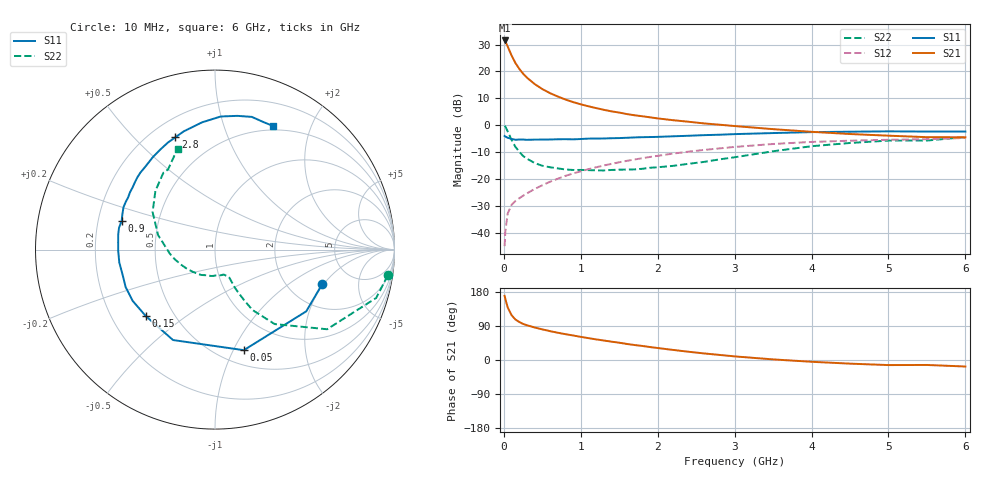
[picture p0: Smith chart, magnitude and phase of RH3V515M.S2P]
! SIEMENS Small Signal Semiconductors
! BFR106
! Si NPN RF Bipolar Junction Transistor in SOT23
! VCE = 3.5 V  IC = 15 mA
! Common Emitter S-Parameters:  August  1996
# GHz  S  MA  R  50
!  f  S11  S21  S12  S22
! GHz  MAG  ANG  MAG  ANG  MAG  ANG  MAG  ANG
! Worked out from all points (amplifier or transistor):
!   36 points, 10 MHz to 6 GHz, reference 50 ohm
!   highest |S21| = 31.5 dB at 10 MHz (marker M1)
!   |S21| within 3 dB of that: start of sweep to 61.44 MHz
!   unconditionally stable (mu >= 1): 413.1 MHz to 2.169 GHz; 5.31 GHz to end of sweep
!   at 250 MHz: K = 0.82, MSG = 22.7 dB, |S12| = -26.3 dB
!   at 1.4 GHz: K = 1.08, MAG = 8.0 dB, |S12| = -14.4 dB
!   at 6 GHz: K = 1.01, MAG = -0.3 dB, |S12| = -4.8 dB
!   S11 on the Smith chart (normalised r, x): 10 MHz: 3.07, -1.93; 50 MHz: 0.65, -1.10; 150 MHz: 0.35, -0.36; 900 MHz: 0.30, +0.14; 2.8 GHz: 0.30, +0.67; 6 GHz: 0.45, +1.47
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0.01  0.6281 -17.6  37.68 169.4  0.0056 84.1  0.9732 -8.5
0.02  0.6138 -34.1  36.13 160.9  0.0107 78.1  0.9376 -16.7
0.05  0.5829 -74.0  29.11 138.8  0.0226 61.1  0.7661 -35.4
0.1  0.5555 -114.9  19.87 118.4  0.0329 52.2  0.5316 -51.3
0.15  0.5346 -136.2  14.37 106.9  0.0388 49.6  0.3958 -58.2
0.2  0.5404 -148.1  11.22 100.4  0.0436 51.3  0.3206 -60.2
0.25  0.5399 -157.3  9.09 95.2  0.0486 53.3  0.2676 -61.6
0.3  0.5338 -163.3  7.66 91.7  0.0538 55.8  0.2383 -62.5
0.4  0.538 -172.3  5.829 85.8  0.0649 58.8  0.1975 -62.7
0.5  0.5392 -179.0  4.692 80.8  0.0761 61.1  0.1755 -62.9
0.6  0.5411 175.7  3.945 76.2  0.0884 62.6  0.1648 -64.4
0.7  0.5459 171.0  3.415 72.0  0.1006 63.4  0.157 -67.2
0.9  0.5442 162.9  2.689 64.7  0.1263 63.4  0.1466 -71.7
1.1  0.5618 155.2  2.243 57.7  0.1517 62.9  0.1457 -80.0
1.3  0.5647 149.0  1.929 51.4  0.1777 61.6  0.1437 -88.1
1.6  0.5826 140.1  1.607 42.3  0.2168 58.8  0.1492 -103.1
2.2  0.6204 124.0  1.237 26.6  0.2957 51.6  0.1748 -134.7
2.8  0.6635 109.4  1.021 13.5  0.3693 42.7  0.2304 -166.5
3.5  0.7127 95.8  0.843 1.6  0.4465 31.7  0.3267 165.8
4.5  0.7555 80.5  0.684 -9.6  0.514 15.7  0.4662 135.4
5.5  0.7598 68.8  0.598 -13.1  0.5473 5.1  0.5171 120.4
6  0.761 65.0  0.594 -17.2  0.5778 -2.4  0.6004 110.3
